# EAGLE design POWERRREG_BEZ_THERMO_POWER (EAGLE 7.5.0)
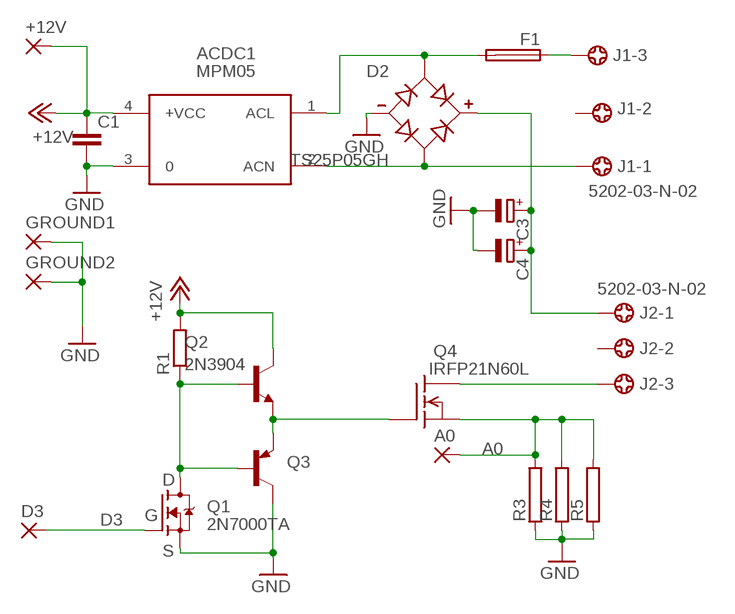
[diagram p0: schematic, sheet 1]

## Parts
+12V  2,54/0,8  [2,54/0,8]
A0  2,54/0,8  [2,54/0,8]
ACDC1  MPM05  [MPM05]
C1  C-EUC1206  [C1206]
C3  CPOL-EUE10-35  [EB35D]
C4  CPOL-EUE10-35  [EB35D]
D2  TS25P05GH  [DIOB_TS25P05GH]
D3  2,54/0,8  [2,54/0,8]
F1  FUSEBLANK_5X20MM  [FUSE_HOLDER_5X20MM]
GROUND1  2,54/0,8  [2,54/0,8]
GROUND2  2,54/0,8  [2,54/0,8]
J1  5202-03-N-02  [5202-03-N-02]
J2  5202-03-N-02  [5202-03-N-02]
Q1  2N7000TA  [TO-92]
Q2  2N3904  [TO92]
Q3  2N3906-PNP-TO92-EBC  [TO92-EBC]
Q4  IRFP21N60L  BUZ325V  [TO218V]
R1  R-EU_R1206  [R1206]
R3  RAC07  [AC07]
R4  RAC07  [AC07]
R5  RAC07  [AC07]

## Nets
+12V: +12V.1(P) ACDC1.4(+VCC) C1.1 Q2.1(C) R1.2
A0: A0.1(P) Q4.3(S) R3.2 R4.2 R5.2
D3: D3.1(P) Q1.2(G)
GND: ACDC1.3 C1.2 C3.- C4.- D2.4(-) GROUND1.1(P) GROUND2.1(P) Q1.1(S) Q3.C R3.1 R4.1 R5.1
N$8: ACDC1.1(ACL) D2.2(AC1) F1.2
N$9: ACDC1.2(ACN) D2.3(AC2) J1.1
N$11: C3.+ C4.+ D2.1(+) J2.1
N$13: J2.3 Q4.2(D)
N$14: Q2.3(E) Q3.E Q4.1(G)
N$16: Q1.3(D) Q2.2(B) Q3.B R1.1
N$19: F1.1 J1.3
Unconnected: J1.2 J2.2

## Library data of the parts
+12V A0 D3 GROUND1 GROUND2 = wirepad:2,54/0,8: THROUGH-HOLE PAD
ACDC1 = acdc:MPM05: AC DC Converter 5W
C1 = rcl:C-EU: CAPACITOR, European symbol
C3 C4 = rcl:CPOL-EU: POLARIZED CAPACITOR, European symbol
D2 = TS25P05GH:TS25P05GH: Check availability; AVAILABILITY: Not in stock; CHECK_PRICES: https://www.snapeda.com/parts/TS25P05GH/taiwan/view-part/?ref=eda; DESCRIPTION: 25A, 600V, Standard Bridge Rectifier; MF: Taiwan Semiconductor; MP: TS25P05GH; PACKAGE: TS-6P Taiwan Semiconductor; PRICE: None; SNAPEDA_LINK: https://www.snapeda.com/parts/TS25P05GH/taiwan/view-part/?ref=snap
F1 = fuse:FUSE: Fuse; OC_FARNELL: unknown; OC_NEWARK: unknown
J1 J2 = con-ebyelectro:5202-03-N-02: Barrier Blocks Sreies 5202 Source: http://www.ebyelectro.com/PDF/5202-XX-N-02.pdf; OC_FARNELL: unknown; OC_NEWARK: unknown
Q1 = 2N7000TA:2N7000TA: http://www.mouser.com/ds/2/149/2N7000TA-347571.pdf Check availability; AVAILABILITY: In Stock; CHECK_PRICES: https://www.snapeda.com/parts/2N7000-TA/Onsemi/view-part/?ref=eda; DESCRIPTION: N-Channel 60 V 200mA (Tc) 400mW (Ta) Through Hole TO-92-3; MF: ON Semiconductor; MP: 2N7000-TA; PACKAGE: E-PKG AXIAL-LEADED-2 ON Semiconductor; PRICE: None; SNAPEDA_LINK: https://www.snapeda.com/parts/2N7000-TA/Onsemi/view-part/?ref=snap
Q2 = transistor-neu-to92:2N3904: NPN TRANSISTOR
Q3 = transistor-neu-to92:*-PNP-: PNP Transistror
Q4 = transistor-fet:BUZ325: N-Channel Enhancement MOSFET 400V; 10,5A; 0,5Ohm
R1 = rcl:R-EU_: RESISTOR, European symbol
R3-R5 = resistor-power:R: Power Resitor; OC_FARNELL: unknown; OC_NEWARK: unknown

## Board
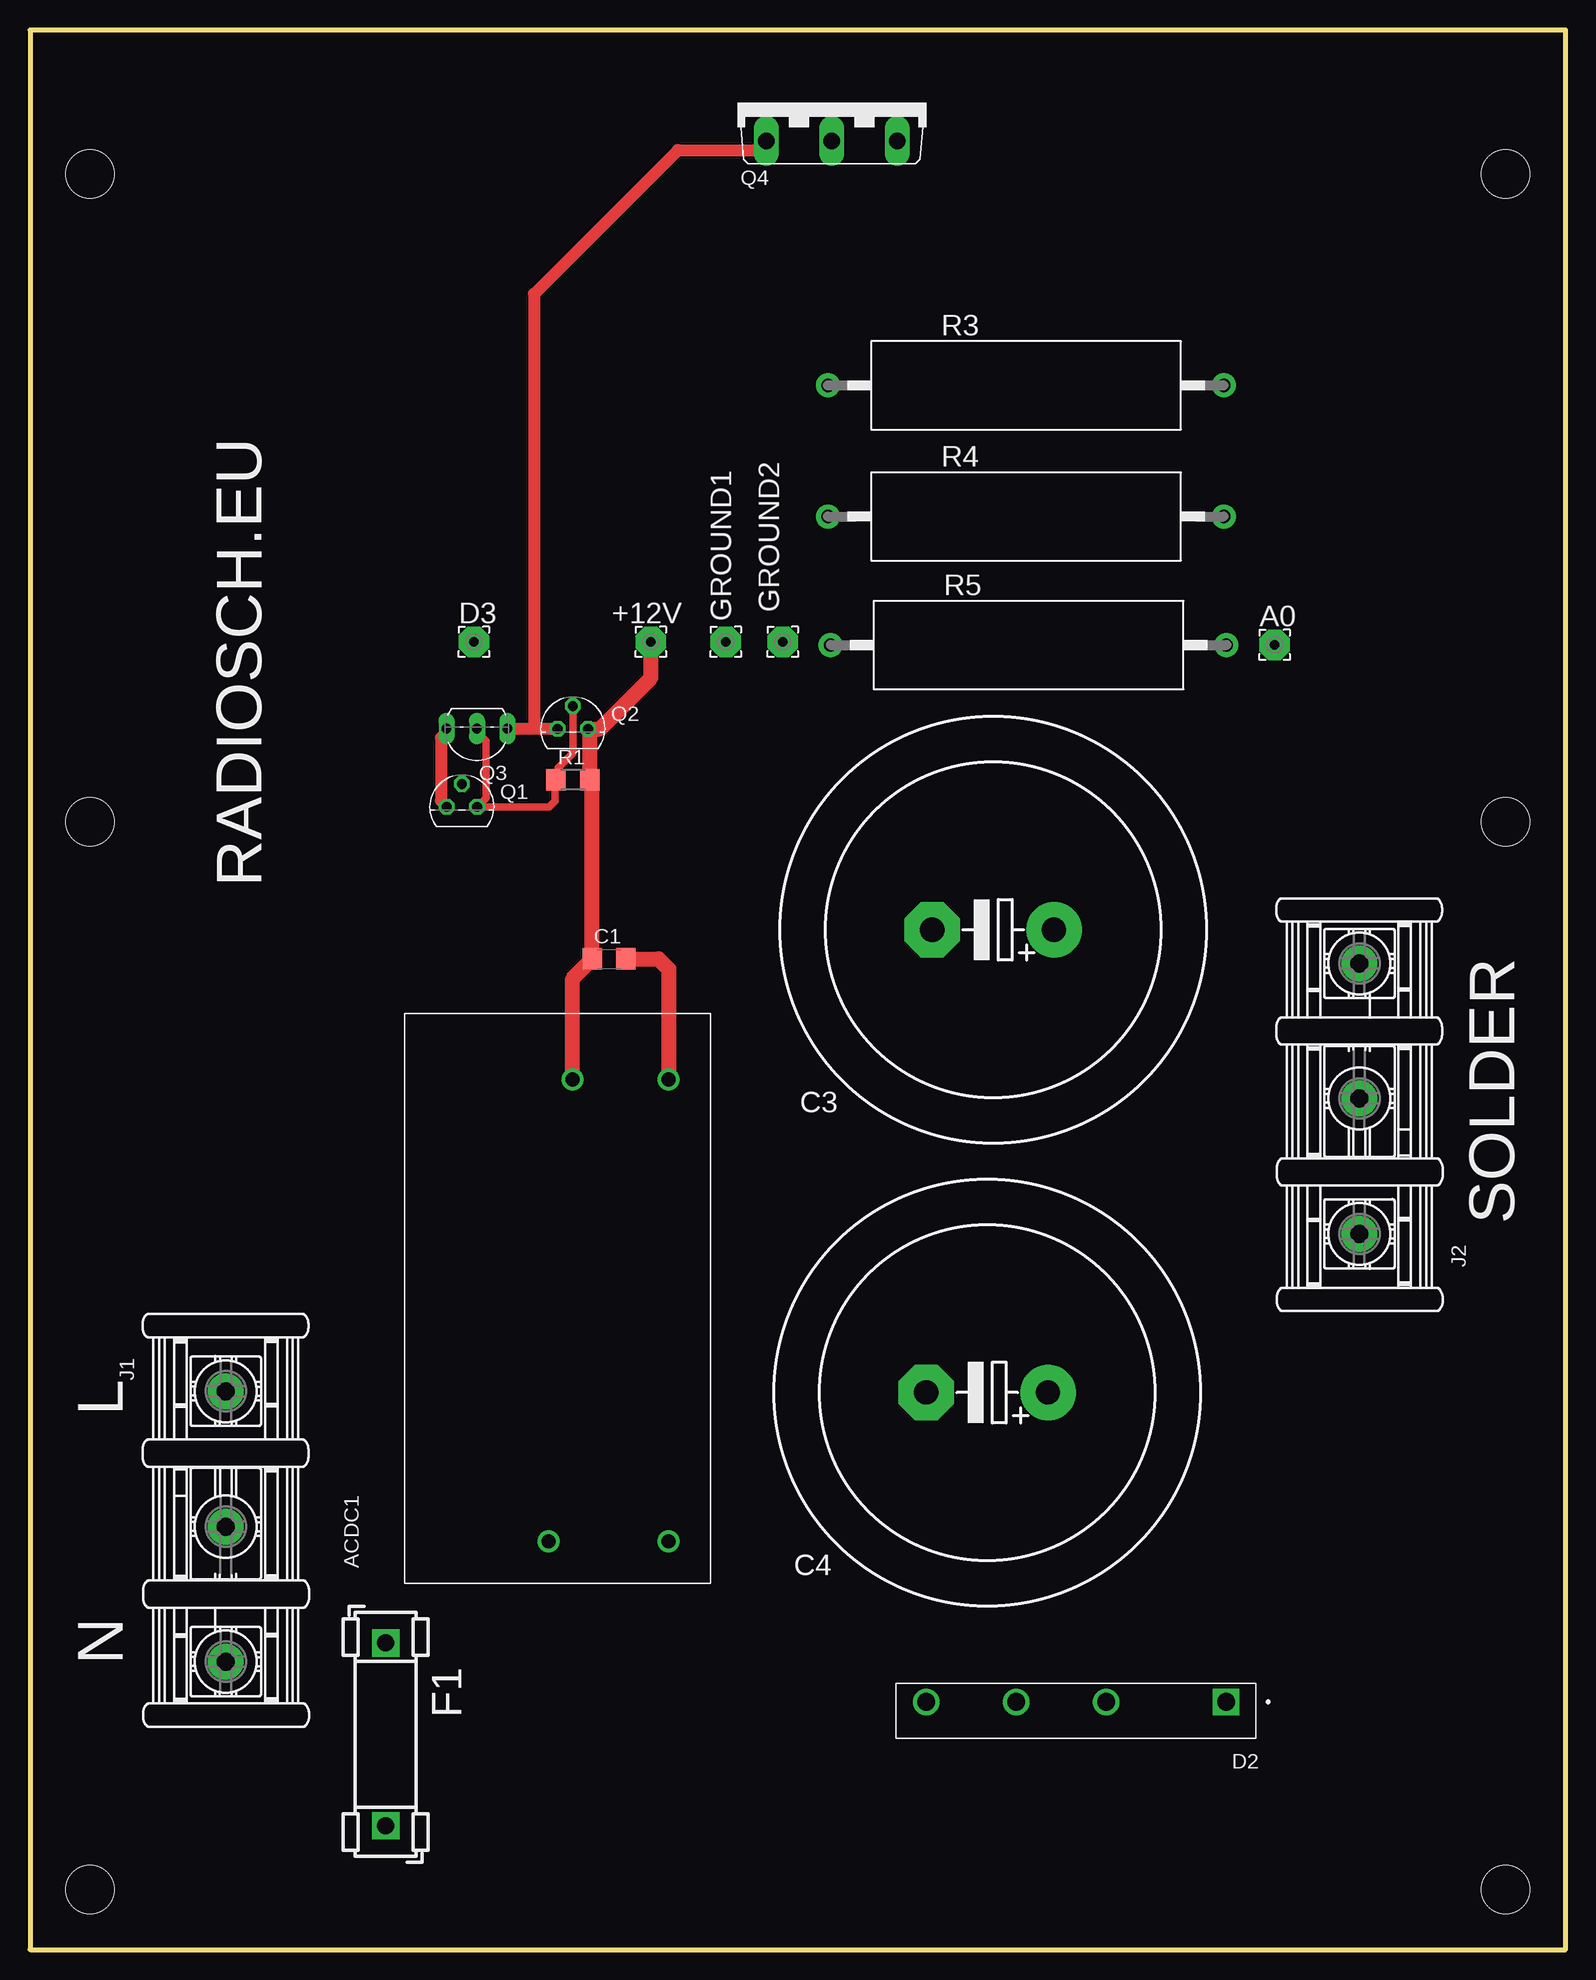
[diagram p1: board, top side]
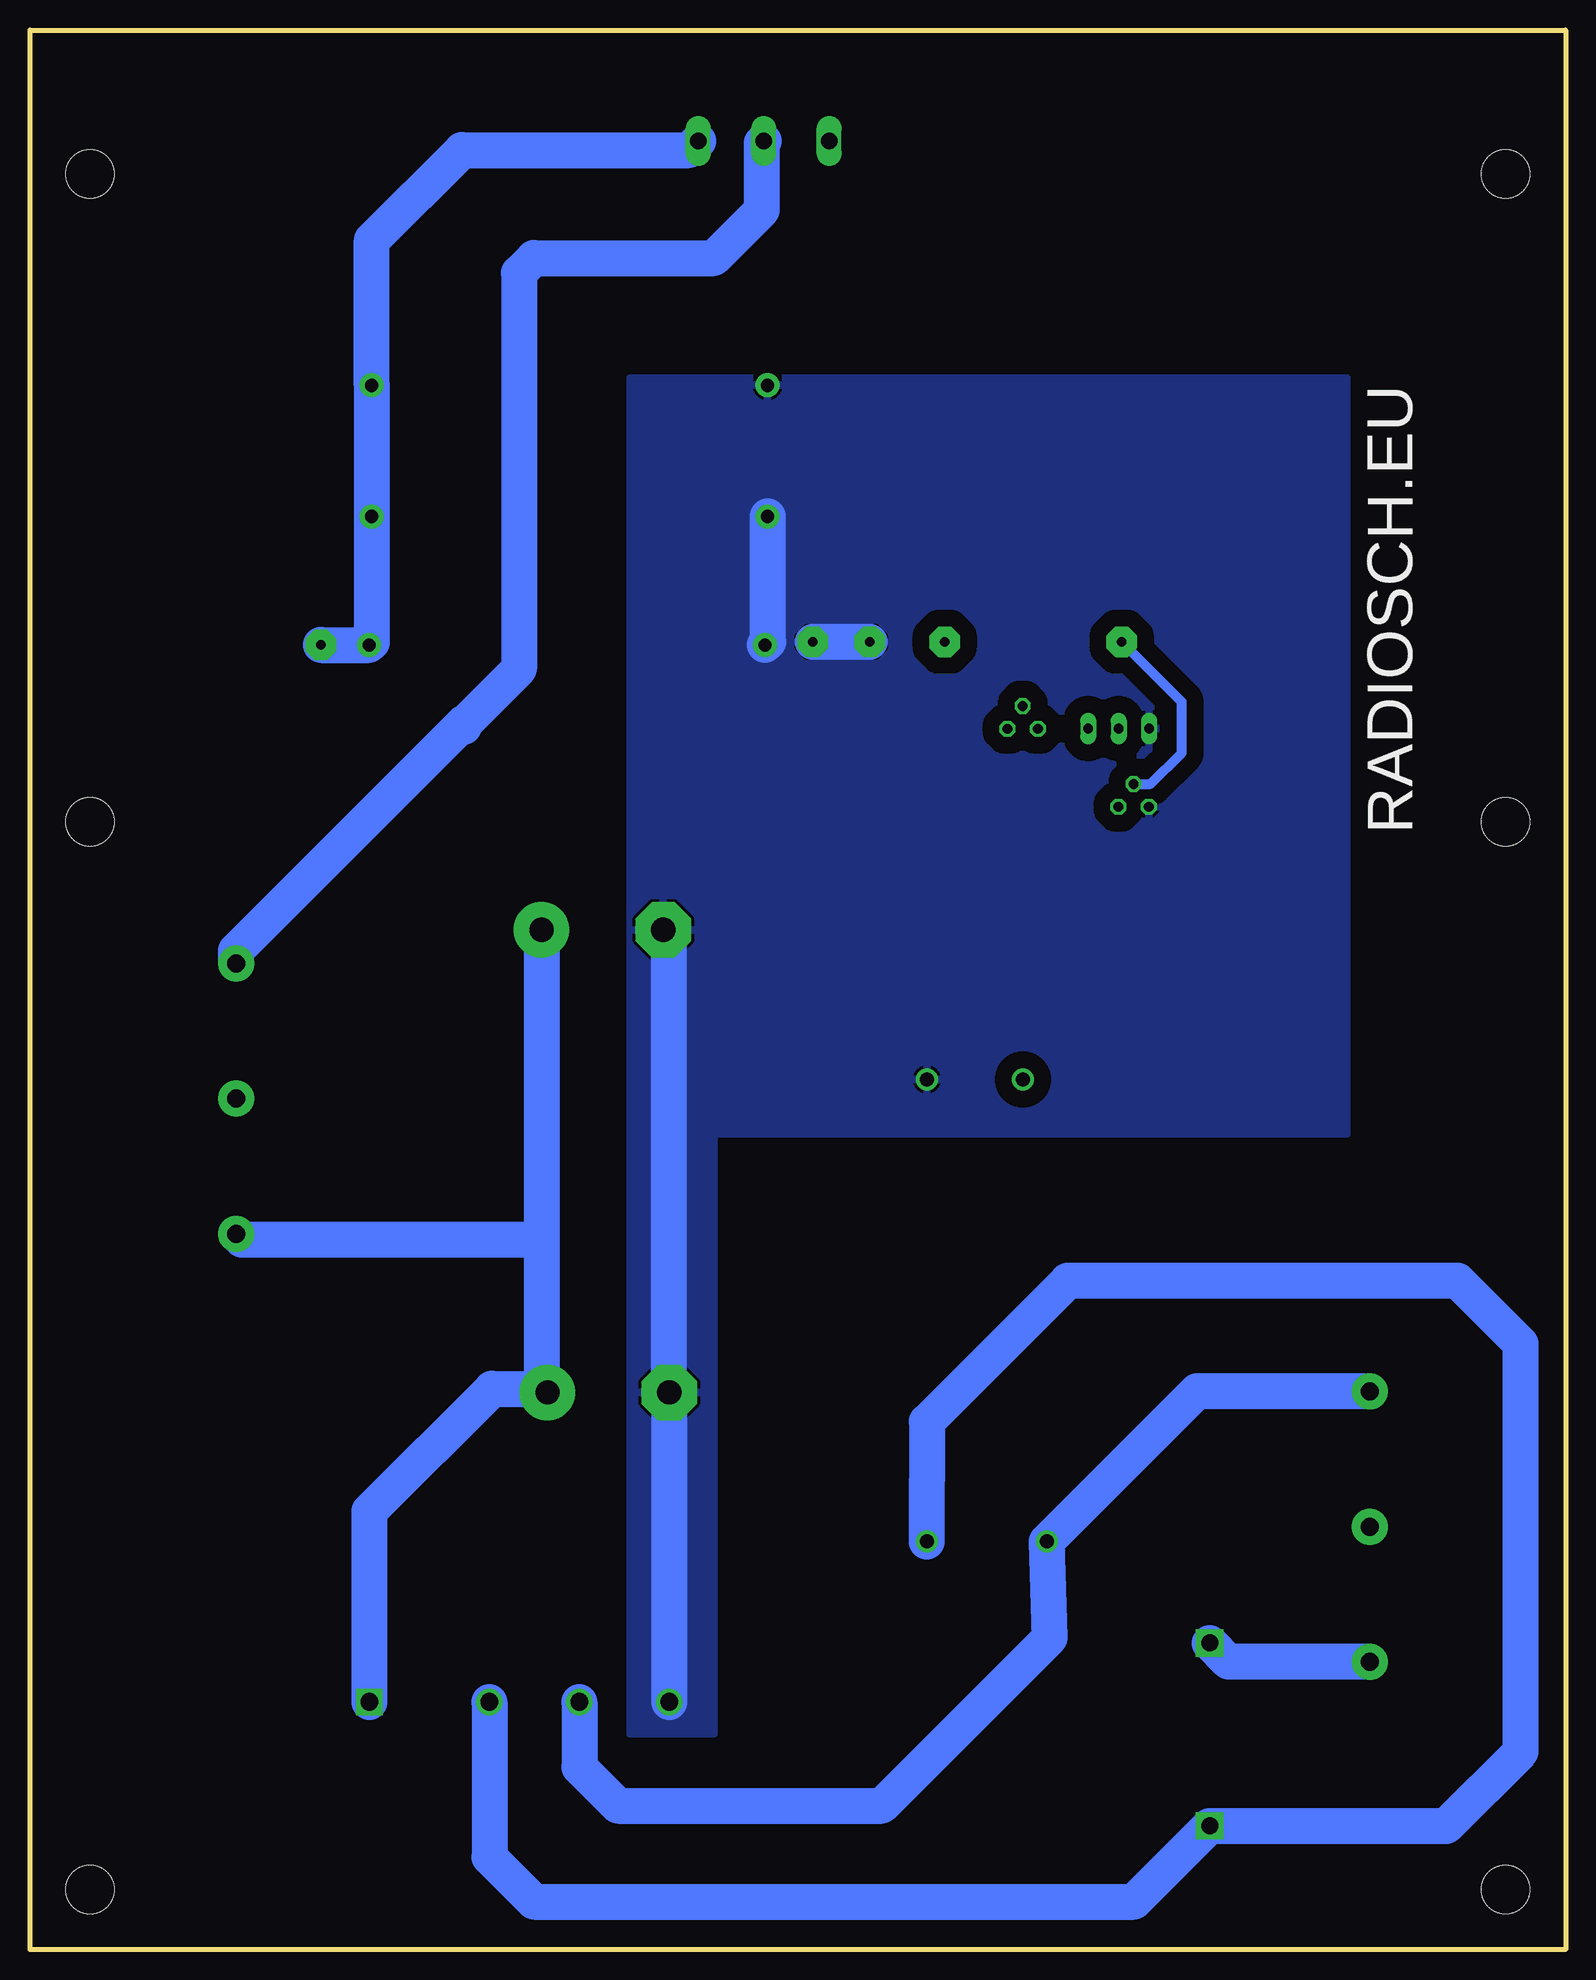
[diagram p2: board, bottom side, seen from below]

Size 128 x 160 mm. Coordinates in mm from the lower left corner, seen from the top.
Outline: 0,0 128,0 128,160 0,160 0,0
Copper layers (1*16): Top 0.035mm / dielectric 1.5mm / Bottom 0.035mm
Design rules "default": minimum track width 10mil, minimum drill 24mil, track to track 8mil, track to pad 8mil, pad to pad 8mil, via to via 8mil, smd to smd 8mil, copper to edge 40mil, drill to drill 8mil, minimum pad ring 10mil, minimum via ring 8mil, stop-mask expansion 4mil, vias tented up to drill 0mil, thermal gap 10mil
Holes 4 mm at 5,5 123,5 5,148 123,148 5,94 123,94

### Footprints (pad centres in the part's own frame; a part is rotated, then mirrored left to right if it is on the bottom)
2,54/0,8 = drill 0.813 pad 2.54 octagon: 1 0,0
MPM05 = drill 1.2: 1 3.5,-22; 2 3.5,-12; 3 42,-22; 4 42,-14
C1206 = smd 1.6 x 1.8: 1 -1.4,0; 2 1.4,0
EB35D = drill 2.007 pad 4.597: + -5.08,0 | drill 2.007 pad 4.597 octagon: - 5.08,0
DIOB_TS25P05GH = drill 1.48 square: 1 0,0 | drill 1.48: 2 10,0; 3 17.5,0; 4 25,0
FUSE_HOLDER_5X20MM = drill 1.422 pad 2.286 square: 1 0,0; 2 15.24,0
5202-03-N-02 = drill 1.5 pad 3: 1 -9.29,0; 2 2,0; 3 13.25,0
TO-92 = drill 0.813 octagon: 1 -1.27,0; 2 0,1.905; 3 1.27,0
TO92 = drill 0.813 octagon: 1 1.27,0; 2 0,1.905; 3 -1.27,0
TO92-EBC = drill 0.813 long: B 0,-1.27; C 2.54,-1.27; E -2.54,-1.27
TO218V = drill 1.397 long: 1 -5.461,-3.175; 2 0,-3.175; 3 5.461,-3.175
R1206 = smd 1.6 x 1.803: 1 -1.422,0; 2 1.422,0
AC07 = drill 1.1 pad 2: 1 -16.5,0; 2 16.5,0

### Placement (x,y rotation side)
+12V  51.75,109 0 top
A0  103.75,108.75 0 top
ACDC1  31.23,30.52 90 top
C1  48.27,82.57 0 top
C3  80.29,85 180 top
C4  79.79,46.42 180 top
D2  99.7,20.64 180 top
D3  37,109 0 top
F1  29.65,25.55 270 top
GROUND1  58,109 0 top
GROUND2  62.75,109 0 top
J1  16.32,37.25 270 top
J2  110.82,68.94 90 top
Q1  36,95.25 0 top
Q2  45.25,101.75 0 top
Q3  37.25,100.5 180 top
Q4  66.84,153.92 0 top
R1  45.25,97.5 0 top
R3  83.02,130.38 0 top
R4  83.02,119.45 0 top
R5  83.23,108.73 0 top

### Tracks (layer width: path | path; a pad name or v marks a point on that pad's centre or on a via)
+12V
  Top 1.27: ACDC1.4 45.23,80.93 C1.1 46.87,97.3 R1.2 46.67,101.6 Q2.1 47.5,101.75 51.75,106 +12V.1
A0
  Bottom 3: A0.1 99.75,108.75 R5.2 99.52,108.94 R4.2 R3.2 99.52,142.48 92,150 73.05,150 Q4.3
D3
  Bottom 0.813: Q1.2 34.59,97.16 32,99.75 32,104 D3.1
GND
  Top 1.016: Q3.C 34.71,101.46 34.25,101 34.25,95.73 Q1.1
  Top 1.27: C1.2 52.41,82.57 53.23,81.75 ACDC1.3
  Bottom 3: C3.- 74.71,84.5 C4.- D2.4 | R4.1 66.52,108.94 R5.1 66.46,109 | GROUND1.1 GROUND2.1
  pour Bottom (isolate 1.422): 78,131 18.25,131 18.25,68 71,68 71,18 78,18
N$8
  Bottom 3: ACDC1.1 53.23,39.02 53.25,39.04 53.25,44 41.5,55.75 9,55.75 3.75,50.5 3.75,16.5 9.94,10.31 F1.2 35.96,4 86,4 89.7,7.7 D2.2
N$9
  Bottom 3: J1.1 30.71,46.54 ACDC1.2 43,26 57,12 79,12 82.2,15.2 D2.3
N$11
  Bottom 3: C3.+ 85.37,59.75 | 85.37,59.75 85.37,47 | 85.37,47 85.37,46.88 85.5,46.75 85.2,46.75 C4.+ | 85.37,59.75 85.97,59.15 110.32,59.15 J2.1 | D2.1 99.7,36.55 89.5,46.75 85.62,46.75 85.37,47
N$13
  Bottom 3: 91.84,102.25 91.84,101.91 | J2.3 110.82,83.27 91.84,102.25 | 91.84,102.25 91.75,102.25 87.25,106.75 87.25,139.75 86,141 71,141 67,145 67,150.59 Q4.2
N$14
  Top 1.016: Q3.E 42,101.77 | 42,101.77 43.96,101.77 Q2.3 | 42,101.77 42,138 54,150 60.63,150 Q4.1
N$16
  Top 0.61: Q2.2 45.25,99.75 44,98.5 44,97.67 R1.1 43.75,97.42 43.75,95.75 43.25,95.25 Q1.3 38,95.98 38,100.75 37.25,101.5 Q3.B
N$19
  Bottom 3: J1.3 28.1,24 F1.1

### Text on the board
tPlace: RADIOSCH.EU | SOLDER | L | N
bPlace: RADIOSCH.EU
